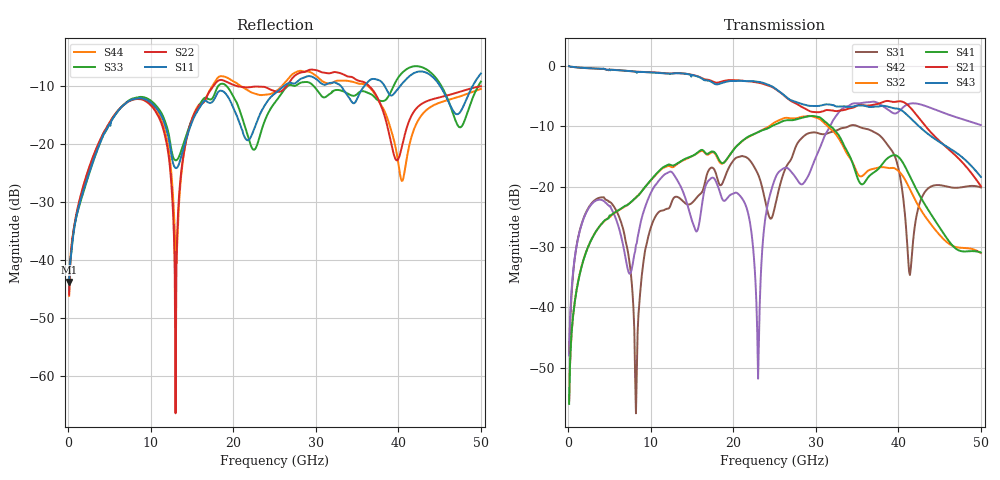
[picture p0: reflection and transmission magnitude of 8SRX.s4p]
! DAC39RF10ACK
! 256-pin FCBGA package
! Texas Instruments 8/20/2022
! Single-ended  S-parameters
! PORT#  PORT_NAME  NET_NAME
! PORT1:  xSRXN.DIEBUMP  xSRXN
! PORT2:  xSRXN.BGA  xSRXN
! PORT3:  xSRXP.DIEBUMP  xSRXP
! PORT4:  xSRXP.BGA  xSRXP
! Touchstone Ver. 1.0
! Number of ports is 4
# Hz	S	MA	R	50.000000
! SCATTERING PARAMETERS  :
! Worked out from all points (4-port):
!   500 points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, 100 MHz to 50 GHz, reference 50 ohm
!   strongest paths, dB at 100 MHz, 12.6 GHz, 25.1 GHz, 37.6 GHz, 50 GHz:
!     S43: 0.0, -1.3, -3.8, -6.7, -18.4
!     S21: -0.1, -1.2, -3.8, -6.3, -19.9
!     S41: -56.0, -16.5, -9.7, -17.0, -30.9
!     S32: -55.5, -16.8, -9.3, -16.8, -31.0
!     S42: -48.0, -17.7, -18.5, -6.2, -9.8
!     S31: -47.9, -22.3, -23.0, -11.4, -20.1
!   lowest |S11| = -43.8 dB at 100 MHz (marker M1), VSWR 1.01, Z = 50.5 + j0.355 ohm
!   |S11| at or under -10 dB: start of sweep to 26.1 GHz; 33.04 GHz to 35.88 GHz (2.836 GHz wide, 8.23 % of centre); 45.06 GHz to 49 GHz (3.937 GHz wide, 8.37 % of centre)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
1e8  0.006434 33.1  0.9946 -2.6  0.004455 78.5  0.00168 -99.9
     0.9916 -2.7  0.005024 35.4  0.001601 -97.4  0.003863 83.2
     0.004035 73.3  0.001673 -100.7  0.005431 41.6  0.9949 -2.6
     0.001583 -95.3  0.003998 81.5  0.9952 -2.6  0.004892 36.7
8e9  0.2444 -67.2  0.8995 -176.1  0.007866 -117.5  0.07891 91.3
     0.8993 -176.5  0.2419 -107.3  0.07919 91.3  0.02671 156.8
     0.006478 -118.1  0.07881 91.8  0.2486 -66.2  0.8972 -175.3
     0.07914 90.9  0.02747 156.3  0.8985 -175.5  0.2464 -106.7
1.3e10  0.06201 -111.6  0.8733 74.9  0.08247 -44.2  0.1527 -22.6
        0.873 74.7  0.0004741 11.1  0.1499 -20.8  0.1189 18.2
        0.08241 -44.1  0.1501 -20.6  0.07232 -110.0  0.871 76.7
        0.1526 -23.0  0.1193 18.4  0.8697 76.7  0.01141 98.0
1.81e10  0.2771 -119.7  0.7296 -36.5  0.1139 56.2  0.1757 -151.1
         0.7266 -36.5  0.3494 -99.3  0.1716 -148.0  0.1015 7.9
         0.1146 55.6  0.1709 -148.0  0.3111 -113.0  0.7047 -33.4
         0.1757 -150.7  0.1019 8.3  0.7042 -33.4  0.3717 -97.4
2.3e10  0.1651 7.0  0.7279 -148.5  0.1266 -64.8  0.2823 113.5
        0.7266 -148.3  0.3125 -133.0  0.2833 118.0  0.002218 16.4
        0.1263 -64.5  0.2826 117.9  0.1042 24.6  0.7386 -143.1
        0.2831 113.9  0.002565 22.9  0.7378 -142.9  0.2665 -135.3
3.31e10  0.3128 -116.8  0.4267 10.6  0.2996 152.6  0.2415 -178.3
         0.4281 10.4  0.4056 -178.4  0.2287 -173.7  0.4351 112.6
         0.3044 152.8  0.2299 -173.5  0.2885 -110.0  0.4614 10.2
         0.2433 -178.8  0.4365 112.7  0.4624 10.3  0.3521 -170.1
5e10  0.4055 -85.7  0.1147 9.0  0.1117 -98.4  0.03609 -119.1
      0.101 10.2  0.3151 -132.3  0.03433 -121.9  0.3379 -27.7
      0.09849 -102.3  0.02817 -104.8  0.3452 -82.3  0.1286 23.2
      0.02845 -97.5  0.3236 -29.0  0.1204 31.9  0.2983 -127.5
